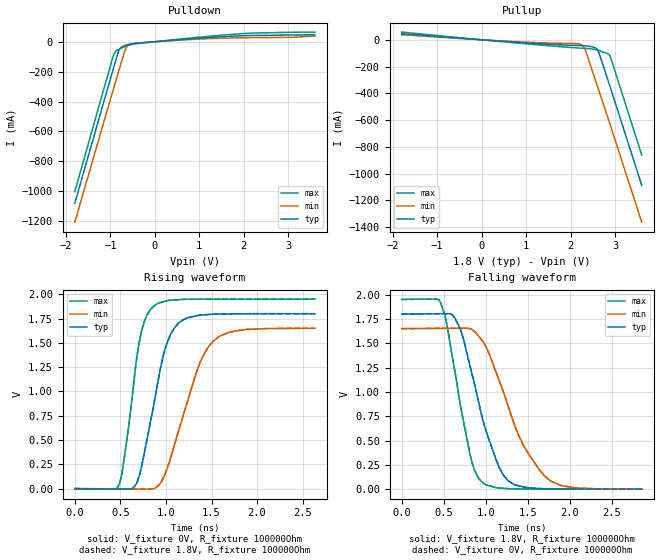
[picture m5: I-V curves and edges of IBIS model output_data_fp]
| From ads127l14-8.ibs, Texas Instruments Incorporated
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|   output_data_fp Model
[Model]   output_data_fp
Model_type   Output
Polarity   Non-Inverting
Vmeas = 0.9
Vref = 0
Cref = 2pF
Rref = 100000
|   typ   min   max
C_comp   0.482pF   0.525pF   0.457pF
[Voltage Range]   1.8   1.65   1.95
[Temperature Range]   27   125   -40
[Pullup Reference]   1.8   1.65   1.95
[Pulldown Reference]   0   0   0
[Power Clamp Reference]   1.8   1.65   1.95
[GND Clamp Reference]   0   0   0
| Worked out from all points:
|   slope of the pulldown table from 0 to 0.27 V, typ, clamps not added: 39.9 ohm
|   slope of the pullup table from 0 to 0.27 V, typ, clamps not added: 41.3 ohm
|   falling waveform, V_fixture 1.8V, R_fixture 100000Ohm: 20-80 % time 335ps typ, 463ps min, 243ps max; typ from 1.8 V to 0.001 V
|   rising waveform, V_fixture 0V, R_fixture 100000Ohm: 20-80 % time 231ps typ, 329ps min, 164ps max; typ from 0 V to 1.8 V
|   rising waveform, V_fixture 1.8V, R_fixture 100000Ohm: 20-80 % time 231ps typ, 329ps min, 164ps max; typ from 0.001 V to 1.8 V
|   falling waveform, V_fixture 0V, R_fixture 100000Ohm: 20-80 % time 335ps typ, 462ps min, 243ps max; typ from 1.8 V to 0 V
[Pulldown]
|   Voltage   I(typ)   I(min)   I(max)
-1.8V     -1.08A     -1.206A    -1.002A
-919.8mV  -167.3mA   -305.9mA   -83.83mA
-876.6mV  -123.3mA   -262.3mA   -62.93mA
-822.6mV  -70.39mA   -207.8mA   -52.24mA
-774mV    -42.33mA   -158.9mA   -45.55mA
-671.4mV  -24.7mA    -59.14mA   -32.58mA
-639mV    -21.9mA    -38.24mA   -28.9mA
-590.4mV  -18.37mA   -21.08mA   -23.98mA
-444.6mV  -11.5mA    -9.365mA   -14.44mA
235.8mV   5.927mA    4.679mA    7.417mA
1.834V    38.58mA    25.73mA    51.49mA
3.6V      46.24mA    38.16mA    64.49mA
[Pullup]
|   Voltage   I(typ)   I(min)   I(max)
-1.8V     45.89mA    37.72mA    57.58mA
765mV     -18.04mA   -13.93mA   -23.34mA
2.131V    -42.16mA   -28.05mA   -60.12mA
2.261V    -43.57mA   -39.89mA   -62.81mA
2.309V    -44.49mA   -60.57mA   -63.75mA
2.358V    -45.9mA    -99.86mA   -64.72mA
2.542V    -58.34mA   -283.8mA   -71.79mA
2.612V    -79.7mA    -354.4mA   -77.48mA
2.639V    -98.78mA   -381.6mA   -80.08mA
2.822V    -284mA     -567.2mA   -101.7mA
2.887V    -350.6mA   -633.1mA   -124.6mA
3.6V      -1.087A    -1.363A    -861.7mA
[Ramp]
R_load = 100000
|   typ   min   max
dV/dt_r   1.07956/2.30213e-10   0.989492/3.28657e-10   1.16963/1.63865e-10
dV/dt_f   1.07958/3.35622e-10   0.989512/4.61896e-10   1.16963/2.41808e-10
[Falling Waveform]
V_fixture = 1.8V
V_fixture_min = 1.65V
V_fixture_max = 1.95V
R_fixture = 100000Ohm
C_fixture = 0F
|   Time   V(typ)   V(min)   V(max)
0s        1.8V       1.65V      1.95V
462.6ps   1.803V     1.652V     1.917V
534.9ps   1.803V     1.653V     1.704V
698.8ps   1.643V     1.653V     861.2mV
839.4ps   1.173V     1.638V     266.5mV
965.1ps   714.6mV    1.519V     66.74mV
1.256ns   96.1mV     880.6mV    6.161mV
1.435ns   26.2mV     473.4mV    2.372mV
1.7ns     3.81mV     135.3mV    816.9uV
2.855ns   815.5uV    930.2uV    681.9uV
[Rising Waveform]
V_fixture = 0V
V_fixture_min = 0V
V_fixture_max = 0V
R_fixture = 100000Ohm
C_fixture = 0F
|   Time   V(typ)   V(min)   V(max)
0s        1.403nV    17.93nV    12.01nV
485.3ps   -3.454mV   -2.947mV   40.26mV
527.5ps   -3.754mV   -3.204mV   213.9mV
714ps     153.4mV    -4.337mV   1.54V
868.3ps   870.7mV    2.055mV    1.879V
980.2ps   1.4V       125.2mV    1.924V
1.088ns   1.646V     431.4mV    1.94V
1.374ns   1.785V     1.296V     1.948V
1.517ns   1.793V     1.515V     1.949V
2.634ns   1.799V     1.649V     1.949V
[Rising Waveform]
V_fixture = 1.8V
V_fixture_min = 1.65V
V_fixture_max = 1.95V
R_fixture = 100000Ohm
C_fixture = 0F
|   Time   V(typ)   V(min)   V(max)
0s        706.9uV    813.3uV    614.2uV
485.3ps   -2.734mV   -2.114mV   40.92mV
527.5ps   -3.034mV   -2.369mV   214.6mV
714ps     154.3mV    -3.494mV   1.541V
868.3ps   871.9mV    2.935mV    1.879V
980.2ps   1.401V     127.8mV    1.927V
1.088ns   1.646V     431.8mV    1.941V
1.366ns   1.785V     1.278V     1.949V
1.51ns    1.794V     1.509V     1.95V
2.634ns   1.8V       1.65V      1.95V
[Falling Waveform]
|Gnd
V_fixture = 0V
V_fixture_min = 0V
V_fixture_max = 0V
R_fixture = 100000Ohm
C_fixture = 0F
|   Time   V(typ)   V(min)   V(max)
0s        1.799V     1.649V     1.949V
462.6ps   1.802V     1.651V     1.916V
534.9ps   1.803V     1.652V     1.703V
698.8ps   1.642V     1.652V     860.3mV
839.4ps   1.172V     1.637V     265.6mV
961.6ps   724.5mV    1.522V     68.5mV
1.256ns   95.22mV    879.1mV    5.542mV
1.445ns   23.49mV    455mV      1.697mV
1.7ns     3.098mV    134mV      202.6uV
2.855ns   108.4uV    116.5uV    67.76uV
